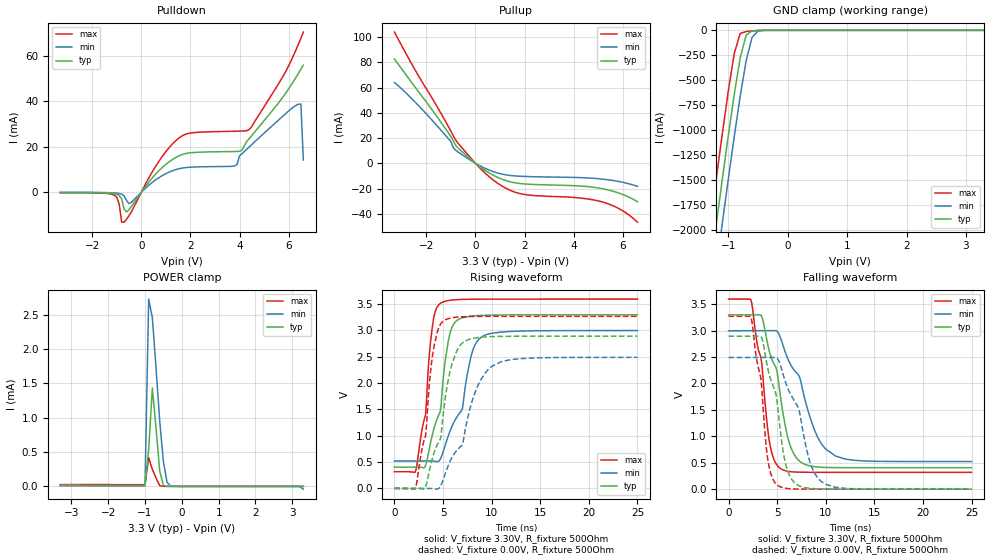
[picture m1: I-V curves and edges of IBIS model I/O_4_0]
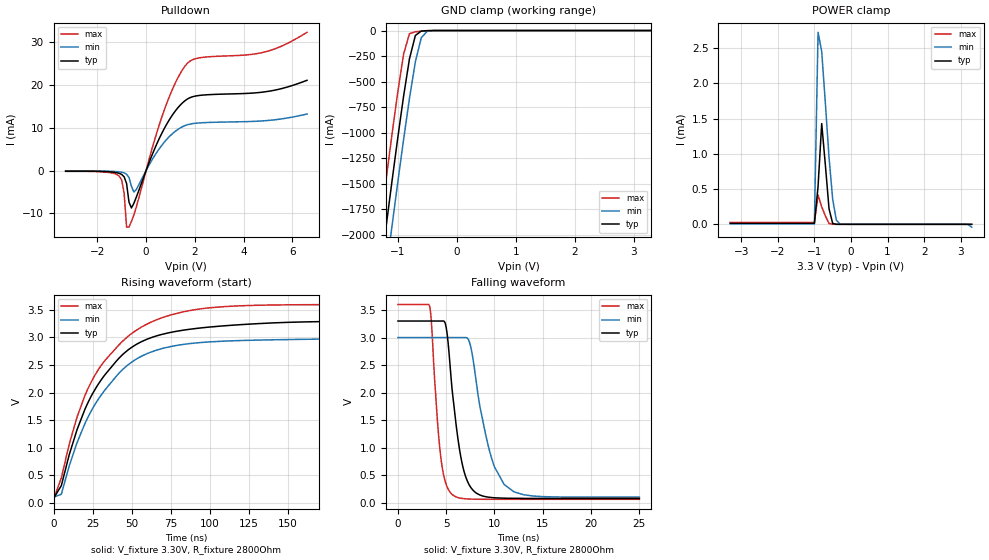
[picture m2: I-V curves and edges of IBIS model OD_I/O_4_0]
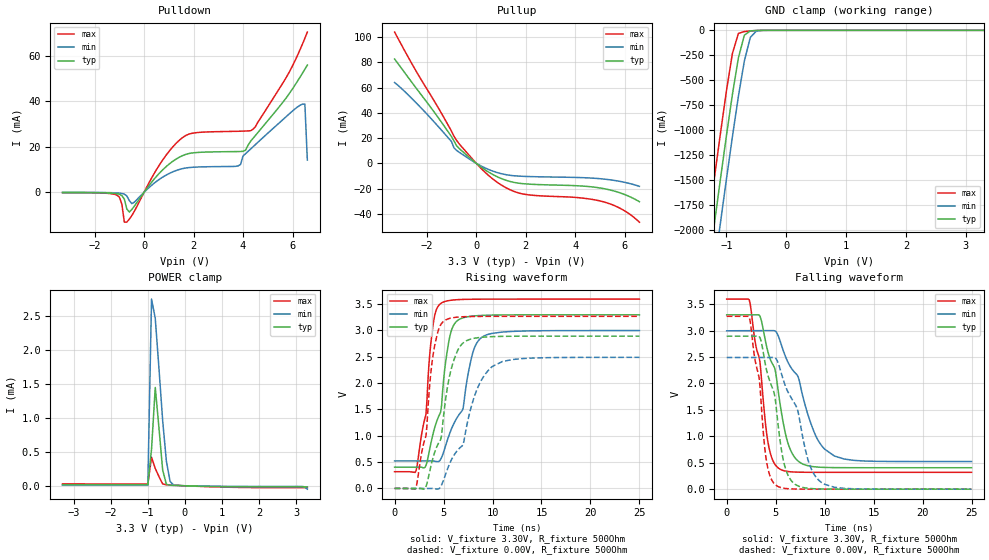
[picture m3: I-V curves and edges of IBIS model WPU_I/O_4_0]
[IBIS Ver]   3.2
[File Name]   lm3s2965_lqfp_v0p1.ibs
[File Rev]   0.1
[Date]   02/19/2010
[Source]   From silicon level SPICE simulations at Texas Instruments
[Notes]   Initial Release of IBIS model
   LM3S2965, Revision A2, 100 LQFP
[Disclaimer] Texas Instruments Confidential - Advance Product Information
   < Software License Agreement >
  Texas Instruments (TI) is supplying this software for use solely and
  exclusively on TI's Stellaris Family of microcontroller products.
  The software is owned by TI and/or its suppliers, and is protected under
  applicable copyright laws.  All rights are reserved.  Any use in violation
  of the foregoing restrictions may subject the user to criminal sanctions
  under applicable laws, as well as to civil liability for the breach of the
  terms and conditions of this license.
  THIS SOFTWARE IS PROVIDED "AS IS".  NO WARRANTIES, WHETHER EXPRESS, IMPLIED
  OR STATUTORY, INCLUDING, BUT NOT LIMITED TO, IMPLIED WARRANTIES OF
  MERCHANTABILITY AND FITNESS FOR A PARTICULAR PURPOSE APPLY TO THIS SOFTWARE.
  LMI SHALL NOT, IN ANY CIRCUMSTANCES, BE LIABLE FOR SPECIAL, INCIDENTAL, OR
  CONSEQUENTIAL DAMAGES, FOR ANY REASON WHATSOEVER.
[Copyright]   Copyright (c) 2010 Texas Instruments.  All rights reserved.
[Component]   LM3S2965 100LQFP
[Manufacturer]  Texas Instruments
[Package]
| 100-pin LQFP
| variable   typ   min   max
R_pkg   125.000m   98.000m   152.000m
L_pkg   7.745nH   6.720nH   8.770nH
C_pkg   0.745pF   0.660pF   0.830pF
[Pin]  signal_name   model_name
   1   ADC0   NC
   2   ADC1   NC
   3   VDDA   POWER
   4   GNDA   GND
   5   ADC2   NC
   6   ADC3   NC
   7   LDO   POWER
   8   VDD   POWER
   9   GND   GND
  10   PD0_CAN0Rx   ProgBuff1
  11   PD1_CAN0Tx   ProgBuff1
  12   PD2_U1Rx   ProgBuff1
  13   PD3_U1Tx   ProgBuff1
  14   VDD25   POWER
  15   GND   GND
  16   PG3_PWM1   ProgBuff2
  17   PG2_PWM0   ProgBuff2
  18   PG1_U2Tx   ProgBuff1
  19   PG0_U2Rx   ProgBuff1
  20   VDD   POWER
  21   GND   GND
  22   PC7   ProgBuff1
  23   PC6   ProgBuff1
  24   PC5   ProgBuff1
  25   PC4_PhA0   ProgBuff1
  26   PA0_U0Rx   ProgBuff1
  27   PA1_U0Tx   ProgBuff1
  28   PA2_SSI0Clk   ProgBuff1
  29   PA3_SSI0Fss   ProgBuff1
  30   PA4_SSI0Rx   ProgBuff1
  31   PA5_SSI0Tx   ProgBuff1
  32   VDD   POWER
  33   GND   GND
  34   PA6_I2C1SCL   ProgBuff1
  35   PA7_I2C1SDA   ProgBuff1
  36   PG7_PhB1   ProgBuff2
  37   PG6_PhA1   ProgBuff2
  38   VDD25   POWER
  39   GND   GND
  40   PG5_CCP5   ProgBuff2
  41   PG4   ProgBuff2
  42   PF7   ProgBuff2
  43   PF6_CCP1   ProgBuff2
  44   VDD   POWER
  45   GND   GND
  46   PF5   ProgBuff2
  47   PF0_CAN1Rx   ProgBuff1
  48   OSC0   NC
  49   OSC1   NC
  50   WAKE   NC
  51   HIB   NC
  52   XOSC0   NC
  53   XOSC1   NC
  54   GND   GND
  55   VBAT   POWER
  56   VDD   POWER
  57   GND   GND
  58   PF4_C0o   ProgBuff1
  59   PF3_PWM5   ProgBuff1
  60   PF2_PWM4   ProgBuff1
  61   PF1_CAN1Tx   ProgBuff1
  62   VDD25   POWER
  63   GND   GND
  64   RST   NC
  65   CMOD0   NC
  66   PB0_CCP0   ProgBuff1
  67   PB1_CCP2   ProgBuff1
  68   VDD   POWER
  69   GND   GND
  70   PB2_I2C0SCL   ProgBuff1
  71   PB3_I2C0SDA   ProgBuff1
  72   PE0_SSI1Clk   ProgBuff1
  73   PE1_SSI1Fss   ProgBuff1
  74   PE2_SSI1Rx   ProgBuff1
  75   PE3_SSI1Tx   ProgBuff1
  76   CMOD1   NC
  77   PC3_TDO_SWO   ProgBuff1
  78   PC2_TDI   ProgBuff1
  79   PC1_TMS_SWDIO   ProgBuff1
  80   PC0_TCK_SWCLK   ProgBuff1
  81   VDD   POWER
  82   GND   GND
  83   PH3_PhB0   ProgBuff2
  84   PH2_IDX1   ProgBuff2
  85   PH1_PWM3   ProgBuff2
  86   PH0_PWM2   ProgBuff2
  87   GND   GND
  88   VDD25   POWER
  89   PB7_TRST   ProgBuff1
  90   PB6   ProgBuff1
  91   PB5   ProgBuff1
  92   PB4   ProgBuff1
  93   VDD   POWER
  94   GND   GND
  95   PD4_CCP3   ProgBuff0
  96   PD5_CCP4   ProgBuff0
  97   GNDA   GND
  98   VDDA   POWER
  99   PD6_Fault   ProgBuff0
 100   PD7_IDX0   ProgBuff0
[Model Selector]   ProgBuff0
I/O_2_0   2 mA buffer without slew rate control
I/O_4_0   4 mA buffer without slew rate control
I/O_8_0   8 mA buffer without slew rate control
I/O_8S_0   8 mA buffer with slew rate control
OD_I/O_2_0   open-drain 2 mA buffer without slew rate control
OD_I/O_4_0   open-drain 4 mA buffer without slew rate control
OD_I/O_8_0   open-drain 8 mA buffer without slew rate control
OD_I/O_8S_0   open-drain 8 mA buffer with slew rate control
WPU_I/O_2_0   weak pullup 2 mA buffer without slew rate control
WPU_I/O_4_0   weak pullup 4 mA buffer without slew rate control
WPU_I/O_8_0   weak pullup 8 mA buffer without slew rate control
WPU_I/O_8S_0   weak pullup 8 mA buffer with slew rate control
WPD_I/O_2_0   weak pulldown 2 mA buffer without slew rate control
WPD_I/O_4_0   weak pulldown 4 mA buffer without slew rate control
WPD_I/O_8_0   weak pulldown 8 mA buffer without slew rate control
WPD_I/O_8S_0   weak pulldown 8 mA buffer with slew rate control
[Model Selector]   ProgBuff1
I/O_2_1   2 mA buffer without slew rate control
I/O_4_1   4 mA buffer without slew rate control
I/O_8_1   8 mA buffer without slew rate control
I/O_8S_1   8 mA buffer with slew rate control
OD_I/O_2_1   open-drain 2 mA buffer without slew rate control
OD_I/O_4_1   open-drain 4 mA buffer without slew rate control
OD_I/O_8_1   open-drain 8 mA buffer without slew rate control
OD_I/O_8S_1   open-drain 8 mA buffer with slew rate control
WPU_I/O_2_1   weak pullup 2 mA buffer without slew rate control
WPU_I/O_4_1   weak pullup 4 mA buffer without slew rate control
WPU_I/O_8_1   weak pullup 8 mA buffer without slew rate control
WPU_I/O_8S_1   weak pullup 8 mA buffer with slew rate control
WPD_I/O_2_1   weak pulldown 2 mA buffer without slew rate control
WPD_I/O_4_1   weak pulldown 4 mA buffer without slew rate control
WPD_I/O_8_1   weak pulldown 8 mA buffer without slew rate control
WPD_I/O_8S_1   weak pulldown 8 mA buffer with slew rate control
[Model Selector]   ProgBuff2
I/O_2_2   2 mA buffer without slew rate control
I/O_4_2   4 mA buffer without slew rate control
I/O_8_2   8 mA buffer without slew rate control
I/O_8S_2   8 mA buffer with slew rate control
OD_I/O_2_2   open-drain 2 mA buffer without slew rate control
OD_I/O_4_2   open-drain 4 mA buffer without slew rate control
OD_I/O_8_2   open-drain 8 mA buffer without slew rate control
OD_I/O_8S_2   open-drain 8 mA buffer with slew rate control
WPU_I/O_2_2   weak pullup 2 mA buffer without slew rate control
WPU_I/O_4_2   weak pullup 4 mA buffer without slew rate control
WPU_I/O_8_2   weak pullup 8 mA buffer without slew rate control
WPU_I/O_8S_2   weak pullup 8 mA buffer with slew rate control
WPD_I/O_2_2   weak pulldown 2 mA buffer without slew rate control
WPD_I/O_4_2   weak pulldown 4 mA buffer without slew rate control
WPD_I/O_8_2   weak pulldown 8 mA buffer without slew rate control
WPD_I/O_8S_2   weak pulldown 8 mA buffer with slew rate control
| Models and submodels in the file (48): I/O_2_0 (I/O), I/O_4_0 (I/O), I/O_8_0 (I/O), I/O_8S_0 (I/O), OD_I/O_2_0 (I/O_open_drain), OD_I/O_4_0 (I/O_open_drain), OD_I/O_8_0 (I/O_open_drain), OD_I/O_8S_0 (I/O_open_drain), WPU_I/O_2_0 (I/O), WPU_I/O_4_0 (I/O), WPU_I/O_8_0 (I/O), WPU_I/O_8S_0 (I/O), WPD_I/O_2_0 (I/O), WPD_I/O_4_0 (I/O), WPD_I/O_8_0 (I/O), WPD_I/O_8S_0 (I/O), I/O_2_1 (I/O), I/O_4_1 (I/O), I/O_8_1 (I/O), I/O_8S_1 (I/O), OD_I/O_2_1 (I/O_open_drain), OD_I/O_4_1 (I/O_open_drain), OD_I/O_8_1 (I/O_open_drain), OD_I/O_8S_1 (I/O_open_drain), WPU_I/O_2_1 (I/O), WPU_I/O_4_1 (I/O), WPU_I/O_8_1 (I/O), WPU_I/O_8S_1 (I/O), WPD_I/O_2_1 (I/O), WPD_I/O_4_1 (I/O), WPD_I/O_8_1 (I/O), WPD_I/O_8S_1 (I/O), I/O_2_2 (I/O), I/O_4_2 (I/O), I/O_8_2 (I/O), I/O_8S_2 (I/O), OD_I/O_2_2 (I/O_open_drain), OD_I/O_4_2 (I/O_open_drain), OD_I/O_8_2 (I/O_open_drain), OD_I/O_8S_2 (I/O_open_drain), WPU_I/O_2_2 (I/O), WPU_I/O_4_2 (I/O), WPU_I/O_8_2 (I/O), WPU_I/O_8S_2 (I/O), WPD_I/O_2_2 (I/O), WPD_I/O_4_2 (I/O), WPD_I/O_8_2 (I/O), WPD_I/O_8S_2 (I/O)
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[Model]   I/O_4_0
Model_type   I/O
Vinl = 1.26
Vinh = 2.04
Vmeas = 1.65
| variable   typ   min   max
C_comp   9.739pF   9.739pF   9.739pF
[Model Spec]
Vinh+   1.91   1.78   2.04
Vinh-   1.90   1.76   2.03
Vinl+   1.40   1.27   1.54
Vinl-   1.39   1.26   1.53
| variable   typ   min   max
[Temperature Range]  25   85   -40
[Voltage Range]   3.3V   3.0V   3.6V
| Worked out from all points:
|   slope of the pulldown table from 0 to 0.495 V, typ, clamps not added: 71.5 ohm
|   slope of the pullup table from 0 to 0.495 V, typ, clamps not added: 71.6 ohm
|   GND clamp passes 1 mA (typ) near -0.48 V on its own axis
|   POWER clamp passes 1 mA (typ) near -0.73 V on its own axis
|   falling waveform, V_fixture 3.30V, R_fixture 500Ohm: 20-80 % time 2.03ns typ, 3.06ns min, 1.36ns max; typ from 3.3 V to 0.405 V
|   rising waveform, V_fixture 3.30V, R_fixture 500Ohm: 20-80 % time 1.61ns typ, 2.31ns min, 1.11ns max; typ from 0.405 V to 3.3 V
|   falling waveform, V_fixture 0.00V, R_fixture 500Ohm: 20-80 % time 1.75ns typ, 2.48ns min, 1.21ns max; typ from 2.89 V to 0 V
|   rising waveform, V_fixture 0.00V, R_fixture 500Ohm: 20-80 % time 1.94ns typ, 2.99ns min, 1.26ns max; typ from 0 V to 2.89 V
[Pulldown]
|  Voltage   I(typ)   I(min)   I(max)
-3.3V     -128.3uA   -72.81uA   -182.3uA
-1.1V     -636.5uA   -293.8uA   -1.284mA
-800mV    -2.996mA   -835.1uA   -13.2mA
-700mV    -7.355mA   -1.607mA   -13.16mA
-500mV    -7.628mA   -5mA       -10.33mA
700mV     9.309mA    6.304mA    13.37mA
1.6V      16.33mA    10.51mA    24.41mA
3.8V      17.94mA    11.61mA    26.87mA
4.4V      23.7mA     20mA       27.72mA
6.4V      52.42mA    38.8mA     65.24mA
6.5V      54.21mA    38.87mA    67.86mA
6.6V      56.01mA    14.21mA    70.56mA
[Pullup]
|  Voltage   I(typ)   I(min)   I(max)
-3.3V     82.57mA    63.94mA    103.9mA
-1.8V     43.25mA    34.86mA    52.68mA
-1V       21.14mA    17.2mA     25.44mA
-900mV    17.77mA    12.26mA    21.52mA
-800mV    14.06mA    10.32mA    18.34mA
100mV     -1.553mA   -1.117mA   -2.117mA
700mV     -9.22mA    -6.424mA   -12.9mA
1.3V      -14.07mA   -9.367mA   -20.37mA
1.9V      -16.2mA    -10.35mA   -24.39mA
5.2V      -20.26mA   -12.6mA    -30.84mA
5.9V      -24.02mA   -14.69mA   -36.54mA
6.6V      -30.45mA   -18.28mA   -46.68mA
[GND Clamp]
|  Voltage   I(typ)   I(min)   I(max)
-3.3V     -11.72A    -12.12A    -11.3A
-1.4V     -2.845A    -3.285A    -2.387A
-1.3V     -2.39A     -2.831A    -1.93A
-1.2V     -1.938A    -2.38A     -1.478A
-1.1V     -1.494A    -1.934A    -1.036A
-1V       -1.059A    -1.496A    -610.6mA
-900mV    -645mA     -1.069A    -232.9mA
-800mV    -277.1mA   -664.4mA   -31.59mA
-700mV    -48.56mA   -306.6mA   -12.09mA
-600mV    -5.558mA   -70.2mA    -6.272mA
-500mV    -1.167mA   -7.88mA    -2.167mA
3.3V      2.282nA    3.101uA    451.3pA
[POWER Clamp]
|  Voltage   I(typ)   I(min)   I(max)
-3.3V     15.18uA    8.315uA    27.48uA
-1V       14.14uA    7.74uA     25.63uA
-900mV    536uA      2.726mA    416.7uA
-800mV    1.43mA     2.454mA    247.6uA
-700mV    840.7uA    1.719mA    119.9uA
-600mV    221.2uA    951.5uA    11.58uA
-500mV    12.35uA    355.6uA    955.3nA
-400mV    305.2nA    58.59uA    44.3nA
-300mV    9.515nA    3.101uA    1.472nA
3.1V      1.302nA    -112.7nA   143.5pA
3.2V      1.207nA    -2.287uA   131.7pA
3.3V      -104.8pA   -40.34uA   119.2pA
[Ramp]
| variable   typ   min   max
dV/dt_f   1.73/2.03n   1.48/3.06n   1.97/1.36n
dV/dt_r   1.74/1.94n   1.49/2.99n   1.96/1.26n
R_load = 500Ohm
[Falling Waveform]
V_fixture = 3.30V
V_fixture_min = 3.00V
V_fixture_max = 3.60V
R_fixture = 500Ohm
|   Time   V(typ)   V(min)   V(max)
0s        3.297V     2.995V     3.595V
2.3ns     3.297V     2.998V     3.582V
3.4ns     3.272V     2.998V     2.405V
4.2ns     2.605V     2.998V     904.6mV
5.3ns     1.806V     2.883V     396.4mV
6.1ns     972.7mV    2.465V     338.6mV
6.9ns     612mV      2.217V     324.2mV
9.1ns     420.8mV    1.008V     318.9mV
11ns      407.6mV    627mV      318.6mV
25ns      405.4mV    522.4mV    318.5mV
[Rising Waveform]
V_fixture = 3.30V
V_fixture_min = 3.00V
V_fixture_max = 3.60V
R_fixture = 500Ohm
|   Time   V(typ)   V(min)   V(max)
0s        405.4mV    522.4mV    318.5mV
2.2ns     405.4mV    522.4mV    343mV
3.2ns     435.5mV    522.4mV    1.4V
3.6ns     760.2mV    522.3mV    2.571V
4ns       1.092V     521.2mV    3.195V
4.7ns     1.449V     551.8mV    3.511V
5.2ns     2.387V     807.4mV    3.554V
5.9ns     3.051V     1.172V     3.578V
9ns       3.287V     2.881V     3.595V
25ns      3.298V     2.999V     3.597V
[Falling Waveform]
V_fixture = 0.00V
V_fixture_min = 0.00V
V_fixture_max = 0.00V
R_fixture = 500Ohm
|   Time   V(typ)   V(min)   V(max)
0s        2.893V     2.49V      3.27V
2.3ns     2.893V     2.491V     3.256V
3.3ns     2.891V     2.491V     2.119V
4.1ns     2.228V     2.491V     489.2mV
5.1ns     1.475V     2.451V     66.08mV
5.7ns     623.9mV    2.118V     22.44mV
6.4ns     215mV      1.79V      7.114mV
8.5ns     13.5mV     445.2mV    479.7uV
9.7ns     3.635mV    124.5mV    177.5uV
25ns      17.27uV    28.07uV    10.86uV
[Rising Waveform]
V_fixture = 0.00V
V_fixture_min = 0.00V
V_fixture_max = 0.00V
R_fixture = 500Ohm
|   Time   V(typ)   V(min)   V(max)
0s        191.9uV    3.961mV    11.2uV
2.2ns     30.29uV    819.6uV    27.43mV
3.2ns     33.68mV    421.3uV    997.8mV
4ns       634.4mV    -846.1uV   2.619V
4.7ns     927.2mV    32.83mV    3.106V
5.1ns     1.54V      213mV      3.188V
6.7ns     2.703V     778mV      3.258V
8.4ns     2.86V      1.876V     3.267V
10ns      2.884V     2.319V     3.269V
25ns      2.893V     2.49V      3.269V
[Model]   OD_I/O_4_0
Model_type   I/O_open_drain
Polarity   Inverting
Vinl = 1.26
Vinh = 2.04
Vmeas = 1.65
Rref = 2800
Vref = 3.3
| variable   typ   min   max
C_comp   9.739pF   9.739pF   9.739pF
[Model Spec]
Vinh+   1.91   1.78   2.04
Vinh-   1.90   1.76   2.03
Vinl+   1.40   1.27   1.54
Vinl-   1.39   1.26   1.53
| variable   typ   min   max
[Temperature Range]  25   85   -40
[Voltage Range]   3.3V   3.0V   3.6V
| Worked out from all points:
|   slope of the pulldown table from 0 to 0.495 V, typ, clamps not added: 71.5 ohm
|   GND clamp passes 1 mA (typ) near -0.48 V on its own axis
|   POWER clamp passes 1 mA (typ) near -0.73 V on its own axis
|   falling waveform, V_fixture 3.30V, R_fixture 2800Ohm: 20-80 % time 1.31ns typ, 2ns min, 884ps max; typ from 3.3 V to 0.075 V
|   rising waveform, V_fixture 3.30V, R_fixture 2800Ohm: 20-80 % time 34.3ns typ, 34ns min, 35.2ns max; typ from 0.075 V to 3.3 V
[Pulldown]
|  Voltage   I(typ)   I(min)   I(max)
-3.3V     -128.3uA   -72.81uA   -182.3uA
-1.1V     -636.5uA   -293.8uA   -1.284mA
-900mV    -1.443mA   -530.4uA   -5.27mA
-800mV    -2.996mA   -835.1uA   -13.2mA
-700mV    -7.355mA   -1.607mA   -13.16mA
-600mV    -8.716mA   -3.66mA    -11.87mA
-500mV    -7.628mA   -5mA       -10.33mA
700mV     9.309mA    6.304mA    13.37mA
1.2V      13.92mA    9.18mA     20.46mA
1.7V      16.72mA    10.71mA    25.07mA
4.9V      18.4mA     11.65mA    27.73mA
6.6V      21.07mA    13.21mA    32.27mA
[GND Clamp]
|  Voltage   I(typ)   I(min)   I(max)
-3.3V     -11.72A    -12.12A    -11.3A
-1.4V     -2.845A    -3.285A    -2.387A
-1.3V     -2.39A     -2.831A    -1.93A
-1.2V     -1.938A    -2.38A     -1.478A
-1.1V     -1.494A    -1.934A    -1.036A
-1V       -1.059A    -1.496A    -610.6mA
-900mV    -645mA     -1.069A    -232.9mA
-800mV    -277.1mA   -664.4mA   -31.59mA
-700mV    -48.56mA   -306.6mA   -12.09mA
-600mV    -5.558mA   -70.2mA    -6.272mA
-500mV    -1.167mA   -7.88mA    -2.167mA
3.3V      2.282nA    3.101uA    451.3pA
[POWER Clamp]
|  Voltage   I(typ)   I(min)   I(max)
-3.3V     15.18uA    8.315uA    27.48uA
-1V       14.14uA    7.74uA     25.63uA
-900mV    536uA      2.726mA    416.7uA
-800mV    1.43mA     2.454mA    247.6uA
-700mV    840.7uA    1.719mA    119.9uA
-600mV    221.2uA    951.5uA    11.58uA
-500mV    12.35uA    355.6uA    955.3nA
-400mV    305.2nA    58.59uA    44.3nA
-300mV    9.515nA    3.101uA    1.472nA
3.1V      1.302nA    -112.7nA   143.5pA
3.2V      1.207nA    -2.287uA   131.7pA
3.3V      -104.8pA   -40.34uA   119.2pA
[Ramp]
| variable   typ   min   max
dV/dt_f   1.93/1.31n   1.74/2.00n   2.12/0.88n
dV/dt_r   1.93/34.25n   1.74/33.99n   2.12/35.16n
R_load = 2800Ohm
[Falling Waveform]
V_fixture = 3.30V
V_fixture_min = 3.00V
V_fixture_max = 3.60V
R_fixture = 2800Ohm
|   Time   V(typ)   V(min)   V(max)
0s        3.3V       2.999V     3.6V
3.3ns     3.3V       2.999V     3.562V
4.4ns     3.3V       2.999V     882.7mV
5ns       3.182V     2.999V     326.2mV
5.7ns     1.912V     2.999V     135.1mV
6.5ns     842.1mV    2.999V     79mV
7.3ns     348.4mV    2.963V     64.72mV
9.4ns     97.23mV    999.2mV    59.1mV
11ns      79.28mV    328.4mV    58.76mV
25ns      75.04mV    97.58mV    58.6mV
[Rising Waveform]
V_fixture = 3.30V
V_fixture_min = 3.00V
V_fixture_max = 3.60V
R_fixture = 2800Ohm
|   Time   V(typ)   V(min)   V(max)
0s        74.96mV    97.48mV    58.55mV
5ns       308.2mV    150.6mV    448mV
10ns      863.6mV    661mV      1.056V
15ns      1.321V     1.084V     1.549V
25ns      1.98V      1.709V     2.238V
43ns      2.655V     2.382V     2.898V
60ns      2.97V      2.708V     3.245V
82ns      3.128V     2.869V     3.459V
110ns     3.214V     2.935V     3.562V
250ns     3.298V     2.994V     3.599V
[Model]   WPU_I/O_4_0
Model_type   I/O
Vinl = 1.26
Vinh = 2.04
Vmeas = 1.65
| variable   typ   min   max
C_comp   9.739pF   9.739pF   9.739pF
[Model Spec]
Vinh+   1.91   1.78   2.04
Vinh-   1.90   1.76   2.03
Vinl+   1.40   1.27   1.54
Vinl-   1.39   1.26   1.53
| variable   typ   min   max
[Temperature Range]  25   85   -40
[Voltage Range]   3.3V   3.0V   3.6V
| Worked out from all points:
|   slope of the pulldown table from 0 to 0.495 V, typ, clamps not added: 71.5 ohm
|   slope of the pullup table from 0 to 0.495 V, typ, clamps not added: 71.7 ohm
|   GND clamp passes 1 mA (typ) near -0.48 V on its own axis
|   POWER clamp passes 1 mA (typ) near -0.73 V on its own axis
|   falling waveform, V_fixture 3.30V, R_fixture 500Ohm: 20-80 % time 2.03ns typ, 3.06ns min, 1.36ns max; typ from 3.3 V to 0.405 V
|   rising waveform, V_fixture 3.30V, R_fixture 500Ohm: 20-80 % time 1.61ns typ, 2.31ns min, 1.11ns max; typ from 0.405 V to 3.3 V
|   falling waveform, V_fixture 0.00V, R_fixture 500Ohm: 20-80 % time 1.75ns typ, 2.48ns min, 1.21ns max; typ from 2.89 V to 0 V
|   rising waveform, V_fixture 0.00V, R_fixture 500Ohm: 20-80 % time 1.94ns typ, 2.99ns min, 1.26ns max; typ from 0 V to 2.89 V
[Pulldown]
|  Voltage   I(typ)   I(min)   I(max)
-3.3V     -128.1uA   -72.69uA   -182uA
-1.1V     -635.5uA   -293.2uA   -1.281mA
-800mV    -2.994mA   -834.1uA   -13.19mA
-700mV    -7.352mA   -1.606mA   -13.14mA
-500mV    -7.614mA   -4.997mA   -10.31mA
700mV     9.325mA    6.314mA    13.4mA
1.6V      16.34mA    10.52mA    24.44mA
3.8V      17.93mA    11.6mA     26.87mA
4.4V      23.7mA     20mA       27.71mA
6.4V      52.42mA    38.8mA     65.24mA
6.5V      54.21mA    38.87mA    67.86mA
6.6V      56.01mA    14.21mA    70.56mA
[Pullup]
|  Voltage   I(typ)   I(min)   I(max)
-3.3V     82.57mA    63.94mA    103.9mA
-1.8V     43.25mA    34.86mA    52.68mA
-1V       21.14mA    17.2mA     25.44mA
-900mV    17.77mA    12.24mA    21.52mA
-800mV    14.04mA    10.31mA    18.34mA
100mV     -1.551mA   -1.116mA   -2.115mA
700mV     -9.21mA    -6.417mA   -12.88mA
1.3V      -14.06mA   -9.358mA   -20.34mA
1.9V      -16.18mA   -10.35mA   -24.37mA
5.2V      -20.25mA   -12.6mA    -30.83mA
5.9V      -24.01mA   -14.69mA   -36.53mA
6.6V      -30.45mA   -18.28mA   -46.68mA
[GND Clamp]
|  Voltage   I(typ)   I(min)   I(max)
-3.3V     -11.72A    -12.12A    -11.3A
-1.4V     -2.845A    -3.285A    -2.387A
-1.3V     -2.39A     -2.831A    -1.93A
-1.2V     -1.938A    -2.38A     -1.478A
-1.1V     -1.494A    -1.934A    -1.036A
-1V       -1.059A    -1.496A    -610.6mA
-900mV    -645mA     -1.069A    -232.9mA
-800mV    -277.1mA   -664.4mA   -31.6mA
-700mV    -48.56mA   -306.6mA   -12.11mA
-600mV    -5.565mA   -70.2mA    -6.295mA
-500mV    -1.181mA   -7.883mA   -2.191mA
3.3V      2.282nA    6.919uA    -6.845uA
[POWER Clamp]
|  Voltage   I(typ)   I(min)   I(max)
-3.3V     15.18uA    8.315uA    27.48uA
-1V       14.14uA    7.74uA     25.63uA
-900mV    539.2uA    2.746mA    419.4uA
-800mV    1.446mA    2.463mA    255uA
-700mV    851uA      1.726mA    135.8uA
-600mV    231.3uA    957.3uA    27.23uA
-500mV    21.69uA    361.2uA    14.14uA
-400mV    7.764uA    63.51uA    10.49uA
-300mV    5.5uA      6.919uA    7.727uA
3.1V      -16.64uA   -9.947uA   -27.43uA
3.2V      -16.65uA   -12.11uA   -27.44uA
3.3V      -16.65uA   -49.87uA   -27.45uA
[Ramp]
| variable   typ   min   max
dV/dt_f   1.73/2.03n   1.48/3.06n   1.97/1.36n
dV/dt_r   1.74/1.94n   1.49/2.99n   1.96/1.26n
R_load = 500Ohm
[Falling Waveform]
V_fixture = 3.30V
V_fixture_min = 3.00V
V_fixture_max = 3.60V
R_fixture = 500Ohm
|   Time   V(typ)   V(min)   V(max)
0s        3.297V     2.995V     3.595V
2.3ns     3.297V     2.998V     3.582V
3.4ns     3.272V     2.998V     2.405V
4.2ns     2.605V     2.998V     904.6mV
5.3ns     1.806V     2.883V     396.4mV
6.1ns     972.7mV    2.465V     338.6mV
6.9ns     612mV      2.217V     324.2mV
9.1ns     420.8mV    1.008V     318.9mV
11ns      407.6mV    627mV      318.6mV
25ns      405.4mV    522.4mV    318.5mV
[Rising Waveform]
V_fixture = 3.30V
V_fixture_min = 3.00V
V_fixture_max = 3.60V
R_fixture = 500Ohm
|   Time   V(typ)   V(min)   V(max)
0s        405.4mV    522.4mV    318.5mV
2.2ns     405.4mV    522.4mV    343mV
3.2ns     435.5mV    522.4mV    1.4V
3.6ns     760.2mV    522.3mV    2.571V
4ns       1.092V     521.2mV    3.195V
4.7ns     1.449V     551.8mV    3.511V
5.2ns     2.387V     807.4mV    3.554V
5.9ns     3.051V     1.172V     3.578V
9ns       3.287V     2.881V     3.595V
25ns      3.298V     2.999V     3.597V
[Falling Waveform]
V_fixture = 0.00V
V_fixture_min = 0.00V
V_fixture_max = 0.00V
R_fixture = 500Ohm
|   Time   V(typ)   V(min)   V(max)
0s        2.893V     2.49V      3.27V
2.3ns     2.893V     2.491V     3.256V
3.3ns     2.891V     2.491V     2.119V
4.1ns     2.228V     2.491V     489.2mV
5.1ns     1.475V     2.451V     66.08mV
5.7ns     623.9mV    2.118V     22.44mV
6.4ns     215mV      1.79V      7.114mV
8.5ns     13.5mV     445.2mV    479.7uV
9.7ns     3.635mV    124.5mV    177.5uV
25ns      17.27uV    28.07uV    10.86uV
[Rising Waveform]
V_fixture = 0.00V
V_fixture_min = 0.00V
V_fixture_max = 0.00V
R_fixture = 500Ohm
|   Time   V(typ)   V(min)   V(max)
0s        192uV      3.962mV    12.12uV
2.2ns     30.3uV     820uV      27.43mV
3.2ns     33.68mV    421.5uV    997.8mV
4ns       634.4mV    -846uV     2.619V
4.7ns     927.2mV    32.83mV    3.106V
5.1ns     1.54V      213mV      3.188V
6.7ns     2.703V     778mV      3.258V
8.4ns     2.86V      1.876V     3.267V
10ns      2.884V     2.319V     3.269V
25ns      2.893V     2.49V      3.269V
